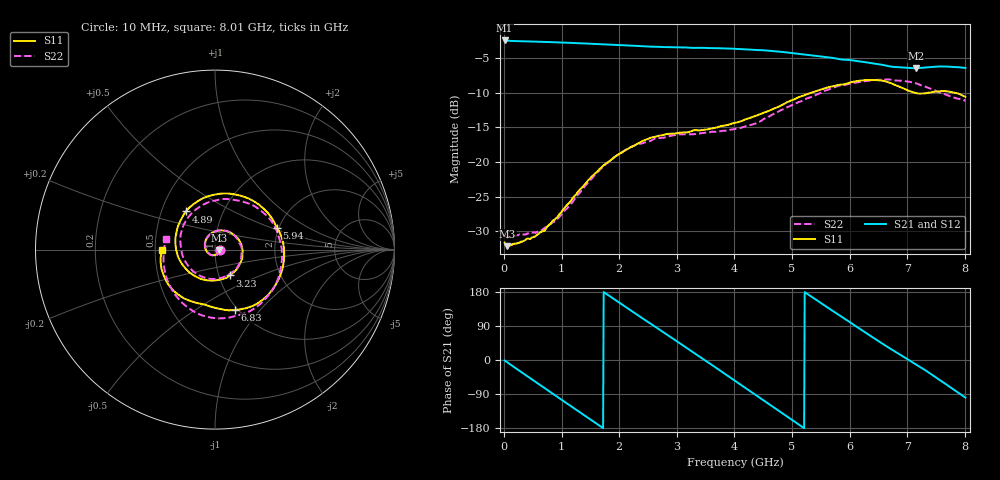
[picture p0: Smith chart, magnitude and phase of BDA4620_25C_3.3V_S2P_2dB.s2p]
!Agilent Technologies,E5071B,MY42404982,A.09.10
!Date: Wed May 06 08:56:23 2026
!Data & Calibration Information:
!Freq	S11:SOLT2(ON)	S21:SOLT2(ON)	S12:SOLT2(ON)	S22:SOLT2(ON)
# Hz S RI R 50
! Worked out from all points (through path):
!   801 points, 10 MHz to 8.01 GHz, reference 50 ohm
!   highest |S21| = -2.44 dB at 10 MHz (marker M1); lowest = -6.5 dB at 7.15 GHz (marker M2)
!   group delay of S21, straight-line fit = 284 ps
!   lowest |S11| = -32.2 dB at 60 MHz (marker M3), VSWR 1.05, Z = 52.5 - j0.402 ohm
!   |S11| at or under -10 dB: start of sweep to 5.328 GHz; 7.132 GHz to 7.371 GHz (239.2 MHz wide, 3.3 % of centre); 7.838 GHz to end of sweep
!   |S22| runs from -30.9 to -8.1 dB; largest |S21 - S12| = 0.0033
!   S11 on the Smith chart (normalised r, x): 10 MHz: 1.05, -0.00; 3.23 GHz: 1.13, -0.33; 4.89 GHz: 0.67, +0.30; 5.94 GHz: 1.95, +0.55; 6.83 GHz: 0.97, -0.75; 8.01 GHz: 0.54, -0.00
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1e7  0.026 -0.00188  0.7549 -0.0163  0.7558 -0.0162  0.0297 -0.00193
6e7  0.0243 -0.00382  0.7468 -0.0864  0.7481 -0.0876  0.0282 -0.00366
3.7e8  0.0178 -0.0206  0.5765 -0.4697  0.577 -0.4713  0.0213 -0.0212
7.3e8  -0.0106 -0.0314  0.1673 -0.7167  0.167 -0.7179  -0.0071 -0.0331
1.03e9  -0.0431 -0.0145  -0.2267 -0.6922  -0.2275 -0.6926  -0.0401 -0.0169
1.35e9  -0.0566 0.0324  -0.563 -0.4487  -0.5631 -0.449  -0.0553 0.0292
1.93e9  0.0242 0.1067  -0.6532 0.2545  -0.654 0.2553  0.0213 0.1072
2.32e9  0.1112 0.0771  -0.3291 0.6051  -0.3304 0.6059  0.1085 0.0783
2.68e9  0.1543 -0.0101  0.0941 0.6724  0.0947 0.6732  0.1485 -0.000965
3.23e9  0.0819 -0.144  0.603 0.2911  0.6043 0.2908  0.0881 -0.132
3.61e9  -0.0272 -0.1726  0.647 -0.1527  0.6479 -0.1531  -0.0189 -0.1643
4.01e9  -0.1476 -0.122  0.3777 -0.5376  0.3776 -0.5386  -0.1361 -0.1072
4.45e9  -0.22 0.0268  -0.1197 -0.6315  -0.1203 -0.6314  -0.1926 0.0399
4.89e9  -0.1619 0.2127  -0.5192 -0.3388  -0.5197 -0.3395  -0.1142 0.2173
5.35e9  0.0611 0.3128  -0.5704 0.1438  -0.5708 0.1441  0.1051 0.2772
5.94e9  0.3452 0.1231  -0.1548 0.5259  -0.154 0.5267  0.3552 0.0706
6.3e9  0.3729 -0.1156  0.1802 0.4916  0.1818 0.4921  0.3567 -0.146
6.68e9  0.2028 -0.3168  0.4153 0.2639  0.4166 0.264  0.2059 -0.3366
6.83e9  0.1114 -0.3364  0.4592 0.1551  0.4602 0.1545  0.1148 -0.3696
7.15e9  -0.0403 -0.3121  0.4662 -0.0943  0.4673 -0.0948  -0.0919 -0.3588
7.63e9  -0.243 -0.2164  0.2482 -0.4219  0.2485 -0.4229  -0.2722 -0.1523
8.01e9  -0.2954 -0.00336  -0.0758 -0.4716  -0.076 -0.4724  -0.2711 0.0591
